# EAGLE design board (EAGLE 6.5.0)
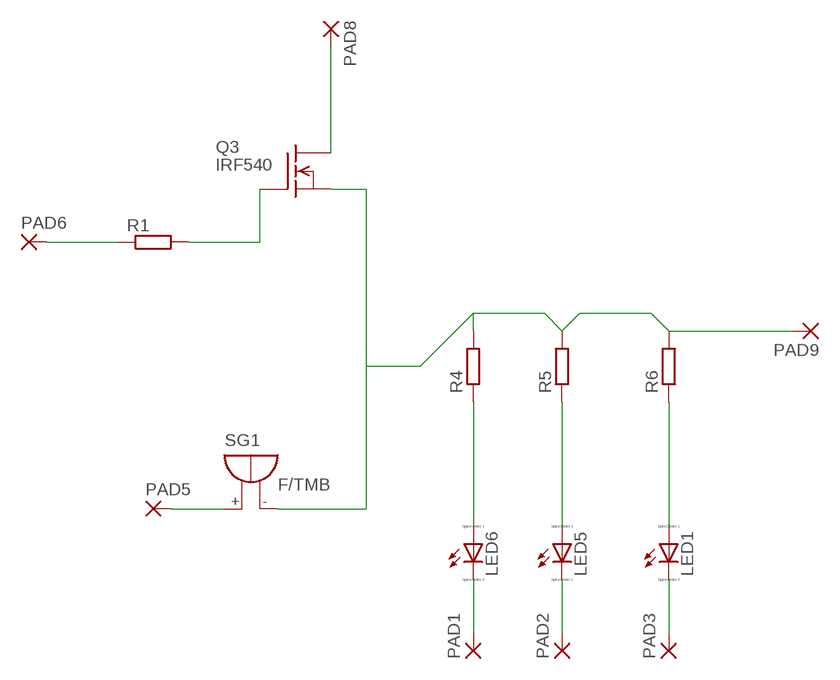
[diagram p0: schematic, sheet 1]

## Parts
LED1  LED_ELD260  [LED_LD260]
LED5  LED_ELD260  [LED_LD260]
LED6  LED_ELD260  [LED_LD260]
PAD1  2,54/1,0  [2,54/1,0]
PAD2  2,54/1,0  [2,54/1,0]
PAD3  2,54/1,0  [2,54/1,0]
PAD5  2,54/1,0  [2,54/1,0]
PAD6  2,54/1,0  [2,54/1,0]
PAD8  2,54/1,0  [2,54/1,0]
PAD9  2,54/1,0  [2,54/1,0]
Q3  IRF540  [TO220]
R1  R-EU_0207/10  [0207/10]
R4  R-EU_0207/10  [0207/10]
R5  R-EU_0207/10  [0207/10]
R6  R-EU_0207/10  [0207/10]
SG1  F/TMB  [F/TMB]

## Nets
N$1: LED6.A R4.1
N$2: LED5.A R5.1
N$3: LED1.A R6.1
N$5: Q3.1(G) R1.2
N$6: PAD6.1(P) R1.1
N$7: LED6.K(C) PAD1.1(P)
N$8: LED5.K(C) PAD2.1(P)
N$9: LED1.K(C) PAD3.1(P)
N$10: PAD5.1(P) SG1.+
N$11: PAD9.1(P) Q3.3(S) R4.2 R5.2 R6.2 SG1.-
N$12: PAD8.1(P) Q3.2(D)

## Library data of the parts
LED1 LED5 LED6 = eagle-ltspice:LED_E: LED; SPICEMODEL: NONE; SPICEPREFIX: D; SPICETYPE: diode
PAD1-PAD3 PAD5 PAD6 PAD8 PAD9 = wirepad:2,54/1,0: THROUGH-HOLE PAD
Q3 = transistor-fet:IRF540: N-Channel Enhancement MOSFET (HEXFET); 100V; 28A; 0,077Ohm
R1 R4-R6 = resistor:R-EU_: RESISTOR, European symbol
SG1 = buzzer:F/TMB: BUZZER; OC_FARNELL: unknown; OC_NEWARK: unknown

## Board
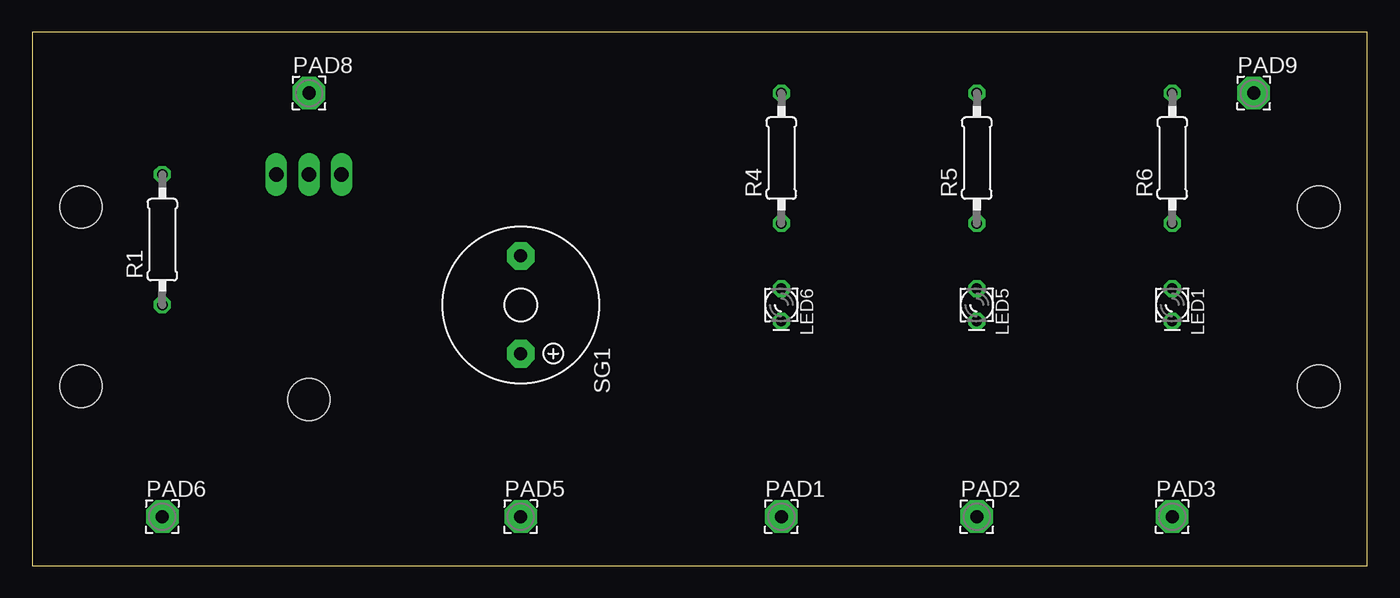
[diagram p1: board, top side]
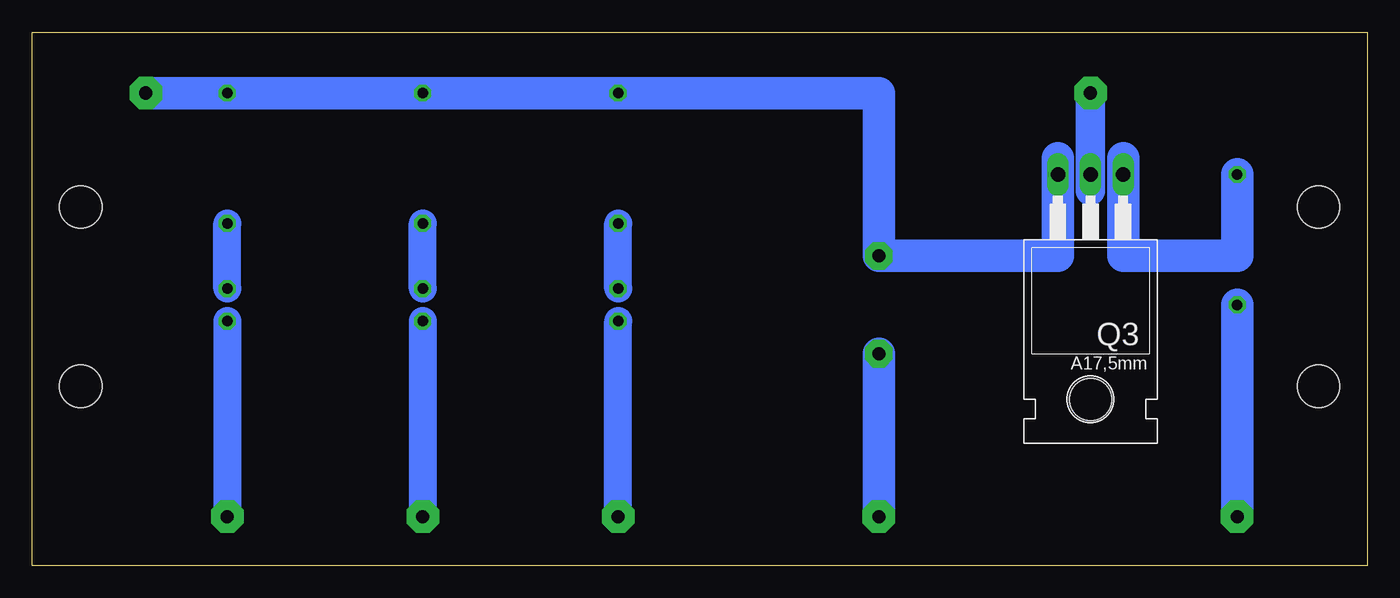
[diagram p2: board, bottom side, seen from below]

Size 104.12 x 41.58 mm. Coordinates in mm from the lower left corner, seen from the top.
Outline: 0,0 104.12,0 104.12,41.58 0,41.58 0,0
Copper layers (1*16): Top 0.035mm / dielectric 1.5mm / Bottom 0.035mm
Design rules "default": minimum track width 10mil, minimum drill 24mil, track to track 8mil, track to pad 8mil, pad to pad 8mil, via to via 8mil, smd to smd 8mil, copper to edge 40mil, drill to drill 8mil, minimum pad ring 10mil, minimum via ring 8mil, stop-mask expansion 4mil, vias tented up to drill 0mil, thermal gap 10mil
Holes 3.3 mm at 3.81,13.97 3.81,27.94 100.33,27.94 100.33,13.97

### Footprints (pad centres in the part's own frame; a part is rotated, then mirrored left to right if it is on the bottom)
LED_LD260 = drill 0.813 octagon: A -1.27,0; K 1.27,0
2,54/1,0 = drill 1.016 pad 2.54 octagon: 1 0,0
TO220 = drill 1.118 long: 1 -2.54,-6.35; 2 0,-6.35; 3 2.54,-6.35 | hole 3.302: 0,11.176
0207/10 = drill 0.813 octagon: 1 -5.08,0; 2 5.08,0
F/TMB = drill 1.016 pad 2.159 octagon: + 3.81,0; - -3.81,0

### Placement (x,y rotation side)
LED1  88.9,20.32 270 top
LED5  73.66,20.32 270 top
LED6  58.42,20.32 270 top
PAD1  58.42,3.81 0 top
PAD2  73.66,3.81 0 top
PAD3  88.9,3.81 0 top
PAD5  38.1,3.81 0 top
PAD6  10.16,3.81 0 top
PAD8  21.59,36.83 0 top
PAD9  95.25,36.83 0 top
Q3  21.59,24.13 180 bottom
R1  10.16,25.4 90 top
R4  58.42,31.75 90 top
R5  73.66,31.75 90 top
R6  88.9,31.75 90 top
SG1  38.1,20.32 270 top

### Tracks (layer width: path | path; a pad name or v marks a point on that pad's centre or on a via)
N$1
  Bottom 2.184: LED6.A R4.1
N$2
  Bottom 2.184: LED5.A R5.1
N$3
  Bottom 2.184: LED1.A R6.1
N$5
  Bottom 2.54: Q3.1 19.05,31.75 19.05,24.13 10.16,24.13 R1.2
N$6
  Bottom 2.54: PAD6.1 R1.1
N$7
  Bottom 2.184: PAD1.1 LED6.K
N$8
  Bottom 2.184: LED5.K PAD2.1
N$9
  Bottom 2.184: LED1.K PAD3.1
N$10
  Bottom 2.54: PAD5.1 SG1.+
N$11
  Bottom 2.54: PAD9.1 R6.2 R5.2 R4.2 38.1,36.83 SG1.- 24.13,24.13 24.13,31.75 Q3.3
N$12
  Bottom 2.286: 21.59,29.21 Q3.2 PAD8.1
